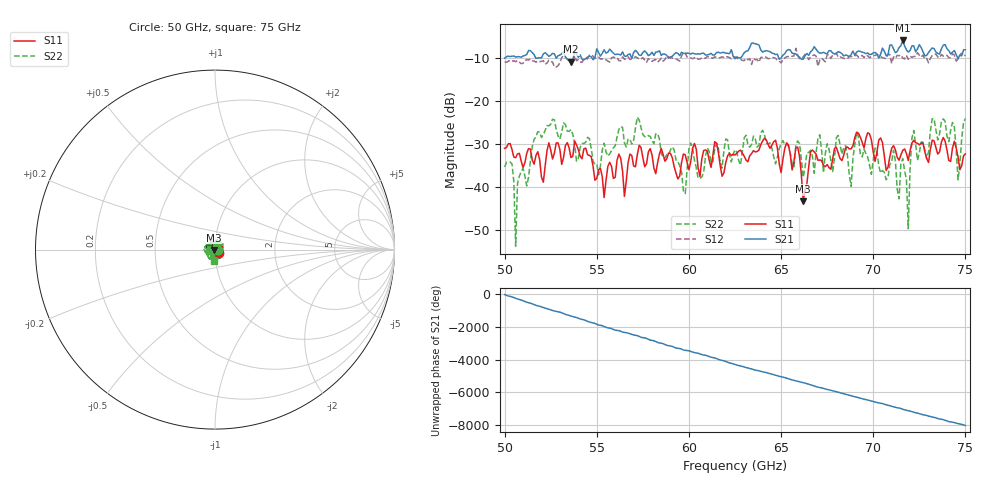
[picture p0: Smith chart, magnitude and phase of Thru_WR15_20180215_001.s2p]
# GHz S RI R 50
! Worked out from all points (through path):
!   251 points, 50 GHz to 75 GHz, reference 50 ohm
!   highest |S21| = -5.97 dB at 71.6 GHz (marker M1); lowest = -10.9 dB at 53.6 GHz (marker M2)
!   lowest |S11| = -43.4 dB at 66.2 GHz (marker M3), VSWR 1.01, Z = 49.3 - j0.139 ohm
!   |S11| at or under -10 dB: start of sweep to end of sweep
!   |S22| runs from -53.9 to -23.8 dB; largest |S21 - S12| = 0.78
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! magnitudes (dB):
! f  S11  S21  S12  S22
! 50 GHz  -31.1  -10.1  -11.0  -35.4
! 50.4 GHz  -31.4  -9.6  -10.8  -34.7
! 50.6 GHz  -33.3  -9.8  -10.9  -53.9
! 50.7 GHz  -32.4  -9.7  -10.7  -39.2
! 51.8 GHz  -31.9  -10.1  -10.8  -27.2
! 53.6 GHz  -33.2  -10.9  -10.6  -26.7
! 54.2 GHz  -33.5  -10.3  -11.1  -29.9
! 56.5 GHz  -42.3  -9.6  -10.3  -29.8
! 58.4 GHz  -32.4  -8.4  -10.6  -28.9
! 59.8 GHz  -32.6  -9.0  -8.9  -41.6
! 60.1 GHz  -34.2  -9.1  -10.0  -29.8
! 62.5 GHz  -32.6  -10.2  -9.8  -31.4
! 65.9 GHz  -30.8  -9.6  -9.3  -29.4
! 66.2 GHz  -43.4  -10.4  -9.8  -37.8
! 66.7 GHz  -31.5  -8.2  -9.5  -33.0
! 70.9 GHz  -33.1  -7.1  -9.3  -34.9
! 71.6 GHz  -31.6  -6.0  -10.1  -33.5
! 71.9 GHz  -33.9  -8.7  -10.4  -49.8
! 72.2 GHz  -29.2  -7.2  -9.7  -26.9
! 74.3 GHz  -31.0  -8.7  -9.1  -25.1
! 74.6 GHz  -33.1  -10.2  -10.3  -38.4
! 75 GHz  -32.4  -8.1  -9.4  -24.1
